|Texas Instruments Incorporated
| 128 Channel, Current-Input Analog-To-Digital Converter
| Marketing part#   Digital Voltage Range   Package-type   #pins
| DDC1128C   2.7V-3.6V   BGA   192
[IBIS Ver]   4.1
[File name]   ddc1128.ibs
[File Rev]   1.0
[Date]   2/14/2014
[Source]
| Texas Instruments Incorporated.
| Analog-eLab Design Center, HPA
| 12500 TI Blvd
| Dallas, TX -75243
[Notes]   Revision History:
| Rev 1.0: 2/14/2014
| - Initial version of the model
| - Model generated from simulations in TISPICE
| - Model matched to SPICE simulation
| - C_comp although listed in numerical order of value are
|   obtained from varying PVT conditions. For PVT conditions for
|   each specific value refer the buffer description under
|   respective [Model]. IBIS model user is responsible for using
|   appropriate C_comp to simulate for Signal Integrity.
[Disclaimer]
| This model is designed as an aid for customers of Texas Instruments.
| TI and its licensors and suppliers make no warranties, either expressed
| or implied, with respect to this  model, including the warranties of
| merchantability or fitness for a particular purpose. The model is
| provided solely on an "as is" basis. The entire risk as to its quality
| and performance is with the customer.
[Copyright]
(C) Copyright 2014 Texas Instruments Incorporated.All rights reserved.
|   DDC1128
[Component]   DDC1128
[Manufacturer]   TI
[Package]   |192 BGA  -  ZKL package
|   typ   min   max
R_pkg   0.00500   0.00500   0.00500
L_pkg   0.20000nH   0.20000nH   0.20000nH
C_pkg   0.60000pF   0.60000pF   0.60000pF
[Pin]  signal_name   model_name   R_pin   L_pin   C_pin
A1   IN120   nc   0.00500   0.20000nH  0.60000pF
A2   IN89   nc   0.00500   0.20000nH  0.60000pF
A3   IN91   nc   0.00500   0.20000nH  0.60000pF
A4   IN92   nc   0.00500   0.20000nH  0.60000pF
A5   IN124   nc   0.00500   0.20000nH  0.60000pF
A6   IN125   nc   0.00500   0.20000nH  0.60000pF
A7   IN126   nc   0.00500   0.20000nH  0.60000pF
A8   IN95   nc   0.00500   0.20000nH  0.60000pF
A9   IN31   nc   0.00500   0.20000nH  0.60000pF
A10   IN128   nc   0.00500   0.20000nH  0.60000pF
A11   IN32   nc   0.00500   0.20000nH  0.60000pF
A12   IN61   nc   0.00500   0.20000nH  0.60000pF
A13   AGND   gnd   0.00500   0.20000nH  0.60000pF
A14   AVDD   power   0.00500   0.20000nH  0.60000pF
A15   AVDD   power   0.00500   0.20000nH  0.60000pF
A16   DVDD   power   0.00500   0.20000nH  0.60000pF
B1   IN88   nc   0.00500   0.20000nH  0.60000pF
B2   IN121   nc   0.00500   0.20000nH  0.60000pF
B3   IN90   nc   0.00500   0.20000nH  0.60000pF
B4   IN27   nc   0.00500   0.20000nH  0.60000pF
B5   IN123   nc   0.00500   0.20000nH  0.60000pF
B6   IN93   nc   0.00500   0.20000nH  0.60000pF
B7   IN94   nc   0.00500   0.20000nH  0.60000pF
B8   IN127   nc   0.00500   0.20000nH  0.60000pF
B9   IN62   nc   0.00500   0.20000nH  0.60000pF
B10   IN63   nc   0.00500   0.20000nH  0.60000pF
B11   IN64   nc   0.00500   0.20000nH  0.60000pF
B12   IN96   nc   0.00500   0.20000nH  0.60000pF
B13   AGND   gnd   0.00500   0.20000nH  0.60000pF
B14   AVDD   power   0.00500   0.20000nH  0.60000pF
B15   AVDD   power   0.00500   0.20000nH  0.60000pF
B16   DGND   gnd   0.00500   0.20000nH  0.60000pF
C1   NC   nc   0.00500   0.20000nH  0.60000pF
C2   NC   nc   0.00500   0.20000nH  0.60000pF
C3   NC   nc   0.00500   0.20000nH  0.60000pF
C4   NC   nc   0.00500   0.20000nH  0.60000pF
C5   NC   nc   0.00500   0.20000nH  0.60000pF
C6   NC   nc   0.00500   0.20000nH  0.60000pF
C7   NC   nc   0.00500   0.20000nH  0.60000pF
C8   NC   nc   0.00500   0.20000nH  0.60000pF
C9   NC   nc   0.00500   0.20000nH  0.60000pF
C10   NC   nc   0.00500   0.20000nH  0.60000pF
C11   NC   nc   0.00500   0.20000nH  0.60000pF
C12   IN30   nc   0.00500   0.20000nH  0.60000pF
C13   AGND   gnd   0.00500   0.20000nH  0.60000pF
C14   AVDD   power   0.00500   0.20000nH  0.60000pF
C15   DIN_CFG   input   0.00500   0.20000nH  0.60000pF
C16   DOUTY   dout   0.00500   0.20000nH  0.60000pF
D1   IN85   nc   0.00500   0.20000nH  0.60000pF
D2   IN117   nc   0.00500   0.20000nH  0.60000pF
D3   IN86   nc   0.00500   0.20000nH  0.60000pF
D4   IN87   nc   0.00500   0.20000nH  0.60000pF
D5   IN119   nc   0.00500   0.20000nH  0.60000pF
D6   IN122   nc   0.00500   0.20000nH  0.60000pF
D7   IN26   nc   0.00500   0.20000nH  0.60000pF
D8   IN58   nc   0.00500   0.20000nH  0.60000pF
D9   IN59   nc   0.00500   0.20000nH  0.60000pF
D10   IN28   nc   0.00500   0.20000nH  0.60000pF
D11   IN29   nc   0.00500   0.20000nH  0.60000pF
D12   IN60   nc   0.00500   0.20000nH  0.60000pF
D13   AGND   gnd   0.00500   0.20000nH  0.60000pF
D14   AVDD   power   0.00500   0.20000nH  0.60000pF
D15   CLK_CFG   input   0.00500   0.20000nH  0.60000pF
D16   DOUTX   dout   0.00500   0.20000nH  0.60000pF
E1   NC   nc   0.00500   0.20000nH  0.60000pF
E2   NC   nc   0.00500   0.20000nH  0.60000pF
E3   NC   nc   0.00500   0.20000nH  0.60000pF
E4   NC   nc   0.00500   0.20000nH  0.60000pF
E5   NC   nc   0.00500   0.20000nH  0.60000pF
E6   NC   nc   0.00500   0.20000nH  0.60000pF
E7   NC   nc   0.00500   0.20000nH  0.60000pF
E8   NC   nc   0.00500   0.20000nH  0.60000pF
E9   NC   nc   0.00500   0.20000nH  0.60000pF
E10   NC   nc   0.00500   0.20000nH  0.60000pF
E11   IN27   nc   0.00500   0.20000nH  0.60000pF
E12   IN25   nc   0.00500   0.20000nH  0.60000pF
E13   AGND   gnd   0.00500   0.20000nH  0.60000pF
E14   AVDD   power   0.00500   0.20000nH  0.60000pF
E15   DGND   gnd   0.00500   0.20000nH  0.60000pF
E16   DINY   din   0.00500   0.20000nH  0.60000pF
F1   IN115   nc   0.00500   0.20000nH  0.60000pF
F2   IN83   nc   0.00500   0.20000nH  0.60000pF
F3   IN114   nc   0.00500   0.20000nH  0.60000pF
F4   IN82   nc   0.00500   0.20000nH  0.60000pF
F5   IN84   nc   0.00500   0.20000nH  0.60000pF
F6   IN116   nc   0.00500   0.20000nH  0.60000pF
F7   IN21   nc   0.00500   0.20000nH  0.60000pF
F8   IN53   nc   0.00500   0.20000nH  0.60000pF
F9   IN22   nc   0.00500   0.20000nH  0.60000pF
F10   IN56   nc   0.00500   0.20000nH  0.60000pF
F11   IN24   nc   0.00500   0.20000nH  0.60000pF
F12   IN55   nc   0.00500   0.20000nH  0.60000pF
F13   AGND   gnd   0.00500   0.20000nH  0.60000pF
F14   AVDD   power   0.00500   0.20000nH  0.60000pF
F15   /RESET   input   0.00500   0.20000nH  0.60000pF
F16   DINX   din   0.00500   0.20000nH  0.60000pF
G1   NC   nc   0.00500   0.20000nH  0.60000pF
G2   NC   nc   0.00500   0.20000nH  0.60000pF
G3   NC   nc   0.00500   0.20000nH  0.60000pF
G4   NC   nc   0.00500   0.20000nH  0.60000pF
G5   NC   nc   0.00500   0.20000nH  0.60000pF
G6   NC   nc   0.00500   0.20000nH  0.60000pF
G7   NC   nc   0.00500   0.20000nH  0.60000pF
G8   NC   nc   0.00500   0.20000nH  0.60000pF
G9   NC   nc   0.00500   0.20000nH  0.60000pF
G10   NC   nc   0.00500   0.20000nH  0.60000pF
G11   NC   nc   0.00500   0.20000nH  0.60000pF
G12   IN23   nc   0.00500   0.20000nH  0.60000pF
G13   AGND   gnd   0.00500   0.20000nH  0.60000pF
G14   AVDD   power   0.00500   0.20000nH  0.60000pF
G15   DGND   gnd   0.00500   0.20000nH  0.60000pF
G16   DCLK   input   0.00500   0.20000nH  0.60000pF
H1   IN81   nc   0.00500   0.20000nH  0.60000pF
H2   IN113   nc   0.00500   0.20000nH  0.60000pF
H3   IN17   nc   0.00500   0.20000nH  0.60000pF
H4   IN49   nc   0.00500   0.20000nH  0.60000pF
H5   IN18   nc   0.00500   0.20000nH  0.60000pF
H6   IN45   nc   0.00500   0.20000nH  0.60000pF
H7   IN54   nc   0.00500   0.20000nH  0.60000pF
H8   IN51   nc   0.00500   0.20000nH  0.60000pF
H9   IN19   nc   0.00500   0.20000nH  0.60000pF
H10   IN20   nc   0.00500   0.20000nH  0.60000pF
H11   IN52   nc   0.00500   0.20000nH  0.60000pF
H12   IN118   nc   0.00500   0.20000nH  0.60000pF
H13   AGND   gnd   0.00500   0.20000nH  0.60000pF
H14   AVDD   power   0.00500   0.20000nH  0.60000pF
H15   DVDD   power   0.00500   0.20000nH  0.60000pF
H16   DVDD   power   0.00500   0.20000nH  0.60000pF
J1   IN80   nc   0.00500   0.20000nH  0.60000pF
J2   IN112   nc   0.00500   0.20000nH  0.60000pF
J3   IN79   nc   0.00500   0.20000nH  0.60000pF
J4   IN111   nc   0.00500   0.20000nH  0.60000pF
J5   IN13   nc   0.00500   0.20000nH  0.60000pF
J6   IN44   nc   0.00500   0.20000nH  0.60000pF
J7   IN14   nc   0.00500   0.20000nH  0.60000pF
J8   IN46   nc   0.00500   0.20000nH  0.60000pF
J9   IN47   nc   0.00500   0.20000nH  0.60000pF
J10   IN15   nc   0.00500   0.20000nH  0.60000pF
J11   IN48   nc   0.00500   0.20000nH  0.60000pF
J12   IN50   nc   0.00500   0.20000nH  0.60000pF
J13   AGND   gnd   0.00500   0.20000nH  0.60000pF
J14   AVDD   power   0.00500   0.20000nH  0.60000pF
J15   DVDD   power   0.00500   0.20000nH  0.60000pF
J16   DVDD   power   0.00500   0.20000nH  0.60000pF
K1   NC   nc   0.00500   0.20000nH  0.60000pF
K2   NC   nc   0.00500   0.20000nH  0.60000pF
K3   NC   nc   0.00500   0.20000nH  0.60000pF
K4   NC   nc   0.00500   0.20000nH  0.60000pF
K5   NC   nc   0.00500   0.20000nH  0.60000pF
K6   NC   nc   0.00500   0.20000nH  0.60000pF
K7   NC   nc   0.00500   0.20000nH  0.60000pF
K8   NC   nc   0.00500   0.20000nH  0.60000pF
K9   NC   nc   0.00500   0.20000nH  0.60000pF
K10   NC   nc   0.00500   0.20000nH  0.60000pF
K11   NC   nc   0.00500   0.20000nH  0.60000pF
K12   IN16   nc   0.00500   0.20000nH  0.60000pF
K13   AGND   gnd   0.00500   0.20000nH  0.60000pF
K14   AVDD   power   0.00500   0.20000nH  0.60000pF
K15   DGND   gnd   0.00500   0.20000nH  0.60000pF
K16   DGND   gnd   0.00500   0.20000nH  0.60000pF
L1   IN78   nc   0.00500   0.20000nH  0.60000pF
L2   IN110   nc   0.00500   0.20000nH  0.60000pF
L3   IN109   nc   0.00500   0.20000nH  0.60000pF
L4   IN77   nc   0.00500   0.20000nH  0.60000pF
L5   IN76   nc   0.00500   0.20000nH  0.60000pF
L6   IN12   nc   0.00500   0.20000nH  0.60000pF
L7   IN108   nc   0.00500   0.20000nH  0.60000pF
L8   IN43   nc   0.00500   0.20000nH  0.60000pF
L9   IN11   nc   0.00500   0.20000nH  0.60000pF
L10   IN42   nc   0.00500   0.20000nH  0.60000pF
L11   IN10   nc   0.00500   0.20000nH  0.60000pF
L12   IN41   nc   0.00500   0.20000nH  0.60000pF
L13   AGND   gnd   0.00500   0.20000nH  0.60000pF
L14   AVDD   power   0.00500   0.20000nH  0.60000pF
L15   DGND   gnd   0.00500   0.20000nH  0.60000pF
L16   CLK   input   0.00500   0.20000nH  0.60000pF
M1   NC   nc   0.00500   0.20000nH  0.60000pF
M2   NC   nc   0.00500   0.20000nH  0.60000pF
M3   NC   nc   0.00500   0.20000nH  0.60000pF
M4   NC   nc   0.00500   0.20000nH  0.60000pF
M5   NC   nc   0.00500   0.20000nH  0.60000pF
M6   NC   nc   0.00500   0.20000nH  0.60000pF
M7   NC   nc   0.00500   0.20000nH  0.60000pF
M8   NC   nc   0.00500   0.20000nH  0.60000pF
M9   NC   nc   0.00500   0.20000nH  0.60000pF
M10   NC   nc   0.00500   0.20000nH  0.60000pF
M11   IN105   nc   0.00500   0.20000nH  0.60000pF
M12   IN9   nc   0.00500   0.20000nH  0.60000pF
M13   AGND   gnd   0.00500   0.20000nH  0.60000pF
M14   AVDD   power   0.00500   0.20000nH  0.60000pF
M15   DGND   gnd   0.00500   0.20000nH  0.60000pF
M16   DVALID   dvalid   0.00500   0.20000nH  0.60000pF
N1   IN75   nc   0.00500   0.20000nH  0.60000pF
N2   IN107   nc   0.00500   0.20000nH  0.60000pF
N3   IN106   nc   0.00500   0.20000nH  0.60000pF
N4   IN74   nc   0.00500   0.20000nH  0.60000pF
N5   IN39   nc   0.00500   0.20000nH  0.60000pF
N6   IN37   nc   0.00500   0.20000nH  0.60000pF
N7   IN5   nc   0.00500   0.20000nH  0.60000pF
N8   IN36   nc   0.00500   0.20000nH  0.60000pF
N9   IN4   nc   0.00500   0.20000nH  0.60000pF
N10   IN40   nc   0.00500   0.20000nH  0.60000pF
N11   IN8   nc   0.00500   0.20000nH  0.60000pF
N12   IN72   nc   0.00500   0.20000nH  0.60000pF
N13   AGND   gnd   0.00500   0.20000nH  0.60000pF
N14   AVDD   power   0.00500   0.20000nH  0.60000pF
N15   DGND   gnd   0.00500   0.20000nH  0.60000pF
N16   DGND   gnd   0.00500   0.20000nH  0.60000pF
P1   NC   nc   0.00500   0.20000nH  0.60000pF
P2   NC   nc   0.00500   0.20000nH  0.60000pF
P3   NC   nc   0.00500   0.20000nH  0.60000pF
P4   NC   nc   0.00500   0.20000nH  0.60000pF
P5   NC   nc   0.00500   0.20000nH  0.60000pF
P6   NC   nc   0.00500   0.20000nH  0.60000pF
P7   NC   nc   0.00500   0.20000nH  0.60000pF
P8   NC   nc   0.00500   0.20000nH  0.60000pF
P9   NC   nc   0.00500   0.20000nH  0.60000pF
P10   NC   nc   0.00500   0.20000nH  0.60000pF
P11   NC   nc   0.00500   0.20000nH  0.60000pF
P12   IN35   nc   0.00500   0.20000nH  0.60000pF
P13   AGND   gnd   0.00500   0.20000nH  0.60000pF
P14   AGND   gnd   0.00500   0.20000nH  0.60000pF
P15   AGND   gnd   0.00500   0.20000nH  0.60000pF
P16   DVDD   power   0.00500   0.20000nH  0.60000pF
R1   IN73   nc   0.00500   0.20000nH  0.60000pF
R2   IN71   nc   0.00500   0.20000nH  0.60000pF
R3   IN104   nc   0.00500   0.20000nH  0.60000pF
R4   IN7   nc   0.00500   0.20000nH  0.60000pF
R5   IN101   nc   0.00500   0.20000nH  0.60000pF
R6   IN100   nc   0.00500   0.20000nH  0.60000pF
R7   IN99   nc   0.00500   0.20000nH  0.60000pF
R8   IN98   nc   0.00500   0.20000nH  0.60000pF
R9   IN6   nc   0.00500   0.20000nH  0.60000pF
R10   IN65   nc   0.00500   0.20000nH  0.60000pF
R11   IN33   nc   0.00500   0.20000nH  0.60000pF
R12   IN34   nc   0.00500   0.20000nH  0.60000pF
R13   QGND   gnd   0.00500   0.20000nH  0.60000pF
R14   VREF   nc   0.00500   0.20000nH  0.60000pF
R15   AGND   gnd   0.00500   0.20000nH  0.60000pF
R16   DGND   gnd   0.00500   0.20000nH  0.60000pF
T1   IN103   nc   0.00500   0.20000nH  0.60000pF
T2   IN70   nc   0.00500   0.20000nH  0.60000pF
T3   IN102   nc   0.00500   0.20000nH  0.60000pF
T4   IN69   nc   0.00500   0.20000nH  0.60000pF
T5   IN68   nc   0.00500   0.20000nH  0.60000pF
T6   IN67   nc   0.00500   0.20000nH  0.60000pF
T7   IN66   nc   0.00500   0.20000nH  0.60000pF
T8   IN97   nc   0.00500   0.20000nH  0.60000pF
T9   IN38   nc   0.00500   0.20000nH  0.60000pF
T10   IN1   nc   0.00500   0.20000nH  0.60000pF
T11   IN2   nc   0.00500   0.20000nH  0.60000pF
T12   IN3   nc   0.00500   0.20000nH  0.60000pF
T13   QGND   gnd   0.00500   0.20000nH  0.60000pF
T14   VREF   nc   0.00500   0.20000nH  0.60000pF
T15   AGND   gnd   0.00500   0.20000nH  0.60000pF
T16   CONV   input   0.00500   0.20000nH  0.60000pF
| Models and submodels in the file (4): input (Input), din (Input), dout (Output), dvalid (Output)
